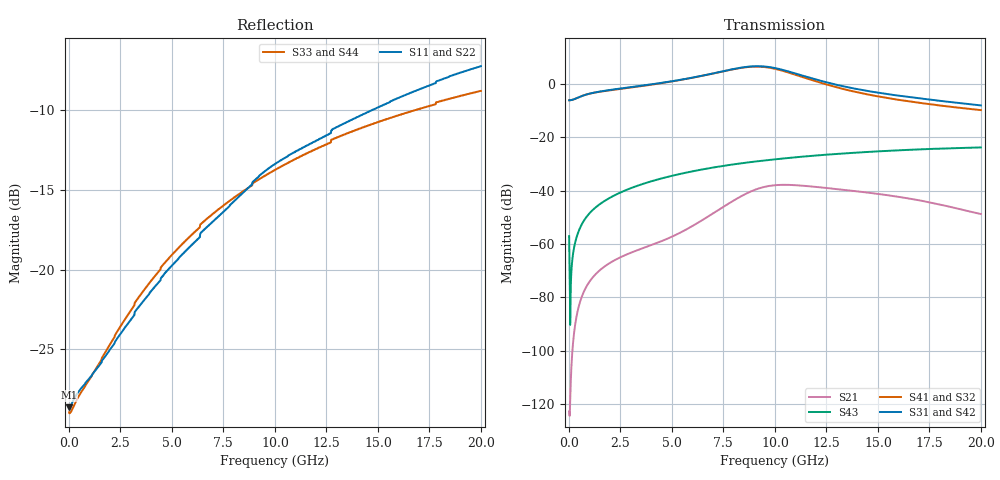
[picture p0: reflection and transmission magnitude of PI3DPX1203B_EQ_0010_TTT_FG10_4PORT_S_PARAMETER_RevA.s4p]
! NPort=4 DATA=2000 NOISE=0 GROUPDELAY=0 COMPLEX_DATAFORMAT=POLAR
! NumOfBlock=1 NumOfParam=0
! .MODEL Smodel S TSTONEFILE=PI3DPX1203B_EQ_0010_TTT_FG10_4PORT_S_PARAMETER_RevA.s4p TYPE=S
!  -- The above .MODEL line can be used for the S element in the netlist.
! The s parameter is extracted from the linear redriver, it is not bi-directional; only s(4,1)s(4,2) and s(3,1)s(3,2)
! should be the insertion loss
!Port definition:
!Port1 = input+
!Port2 = input-
!Port3 = output+
!Port4 = output-
# Hz S MA R  50
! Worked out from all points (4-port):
!   2000 points, 10 MHz to 20 GHz, reference 50 ohm
!   strongest paths, dB at 10 MHz, 5.01 GHz, 10.01 GHz, 15.01 GHz, 20 GHz:
!     S31: -6.2, 1.0, 5.9, -3.3, -8.1
!     S42: -6.2, 1.0, 5.9, -3.3, -8.1
!     S41: -6.2, 0.9, 5.6, -4.7, -9.9
!     S32: -6.2, 0.9, 5.6, -4.7, -9.8
!     S43: -57.1, -34.4, -28.3, -25.3, -23.8
!     S21: -122.7, -57.2, -38.0, -41.2, -48.8
!   lowest |S11| = -28.6 dB at 10 MHz (marker M1), VSWR 1.08, Z = 46.4 - j0.0306 ohm
!   |S11| at or under -10 dB: start of sweep to 14.7 GHz
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1e7  0.03701 -179.5  7.338e-07 10.5  0 0.0  0 0.0
     7.338e-07 10.5  0.03701 -179.5  0 0.0  0 0.0
     0.4917 -0.1  0.4917 179.9  0.03566 178.2  0.001403 -77.8
     0.4917 179.9  0.4917 -0.1  0.001403 -77.8  0.03566 178.2
1.58e9  0.05108 -144.6  0.0003426 113.6  5.327e-12 74.9  5.087e-11 115.5
        0.0003426 113.6  0.05108 -144.6  5.087e-11 115.5  5.327e-12 74.9
        0.7244 1.2  0.7177 -178.8  0.05212 -142.0  0.005859 82.8
        0.7177 -178.8  0.7244 1.2  0.005859 82.8  0.05212 -142.0
6.19e9  0.1235 -111.2  0.002403 130.0  1.708e-08 -111.5  1.585e-07 66.2
        0.002404 130.0  0.1235 -111.2  1.584e-07 66.2  1.708e-08 -111.4
        1.348 -49.2  1.342 133.2  0.1326 -116.9  0.02375 64.3
        1.342 133.2  1.348 -49.2  0.02375 64.3  0.1326 -116.9
8.65e9  0.1791 -106.2  0.008947 103.1  4.306e-07 159.2  1.204e-06 16.2
        0.008943 103.1  0.1791 -106.2  1.202e-06 16.2  4.305e-07 159.2
        2.081 -102.2  2.052 79.8  0.1795 -115.9  0.03355 51.6
        2.053 79.8  2.08 -102.2  0.03355 51.6  0.1795 -115.9
1.01e10  0.2167 -107.4  0.01271 61.0  1.342e-06 96.6  2.338e-06 -21.7
         0.01271 61.0  0.2166 -107.4  2.334e-06 -21.6  1.342e-06 96.7
         1.936 -149.0  1.868 32.8  0.2074 -116.3  0.03884 43.8
         1.87 32.8  1.934 -149.0  0.03884 43.8  0.2074 -116.3
1.221e10  0.258 -108.7  0.01149 17.7  3.174e-06 31.1  4.137e-06 -49.6
          0.0115 17.8  0.258 -108.6  4.137e-06 -49.4  3.175e-06 31.1
          1.142 167.2  1.047 -10.2  0.2425 -117.6  0.04612 33.1
          1.048 -10.2  1.141 167.3  0.04612 33.1  0.2425 -117.6
2e10  0.4349 -116.5  0.003614 -29.4  2.188e-05 -106.1  3.26e-05 -134.0
      0.003645 -29.8  0.435 -116.5  3.269e-05 -134.0  2.191e-05 -106.0
      0.3938 85.7  0.3223 -75.3  0.3637 -123.9  0.06431 -7.1
      0.3216 -75.4  0.3943 85.8  0.06431 -7.1  0.3637 -123.9
